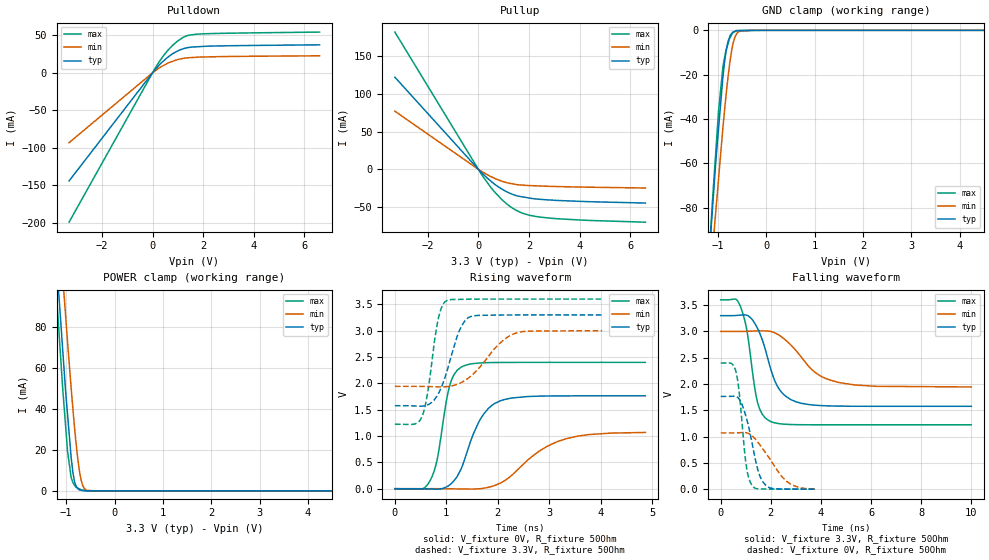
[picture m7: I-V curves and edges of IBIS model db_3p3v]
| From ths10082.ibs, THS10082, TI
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|   db_3p3v Model
[Model]   db_3p3v
Model_type   I/O
Polarity   Non-Inverting
Enable   Active-High
Vinl = 0.6
Vinh = 2
Vmeas = 1.65
Vref = 1.65
Cref = 30pF
Rref = 50
|   typ   min   max
C_comp   1.842e-12   1.833e-12   1.884e-12
[Voltage Range]   3.3   3   3.6
|Ambient Temperature   25   85   -40
|Junction Temperature
[Temperature Range]   27   125   -40
[Pullup Reference]   3.3   3   3.6
[Pulldown Reference]   0   0   0
[Power Clamp Reference]   3.3   3   3.6
[GND Clamp Reference]   0   0   0
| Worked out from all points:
|   slope of the pulldown table from 0 to 0.495 V, typ, clamps not added: 28 ohm
|   slope of the pullup table from 0 to 0.495 V, typ, clamps not added: 31.6 ohm
|   GND clamp passes 1 mA (typ) near -0.70 V on its own axis
|   POWER clamp passes 1 mA (typ) near -0.75 V on its own axis
|   falling waveform, V_fixture 3.3V, R_fixture 50Ohm: 20-80 % time 742ps typ, 1.28ns min, 446ps max; typ from 3.3 V to 1.58 V
|   rising waveform, V_fixture 0V, R_fixture 50Ohm: 20-80 % time 447ps typ, 848ps min, 252ps max; typ from 0 V to 1.76 V
|   rising waveform, V_fixture 3.3V, R_fixture 50Ohm: 20-80 % time 334ps typ, 575ps min, 209ps max; typ from 1.58 V to 3.3 V
|   falling waveform, V_fixture 0V, R_fixture 50Ohm: 20-80 % time 501ps typ, 943ps min, 292ps max; typ from 1.76 V to 0 V
[Pulldown]
|   Voltage   I(typ)   I(min)   I(max)
-3.3V     -144.5mA   -93.38mA   -199.6mA
154.8mV   6.391mA    3.9mA      9.041mA
424.8mV   15.59mA    9.622mA    22.52mA
630mV     21.64mA    13.42mA    30.96mA
1.008V    29.35mA    17.89mA    42.82mA
1.35V     33.32mA    19.96mA    49.36mA
1.836V    34.94mA    21.01mA    51.79mA
6.6V      37.38mA    22.72mA    54.4mA
[GND Clamp]
|   Voltage   I(typ)   I(min)   I(max)
-3.3V     -897.7mA   -838.9mA   -975.7mA
-1.234V   -118.3mA   -135.3mA   -121.5mA
-1.12V    -83.01mA   -102.4mA   -79.59mA
-1.065V   -66.19mA   -87.36mA   -61.92mA
-986.4mV  -44.52mA   -67.16mA   -36.62mA
-896.4mV  -21.17mA   -44.06mA   -16.6mA
-825mV    -8.688mA   -28.04mA   -8.718mA
-788.7mV  -4.936mA   -20.89mA   -5.997mA
-711mV    -1.339mA   -8.661mA   -1.849mA
-620.4mV  -156.6uA   -1.912mA   -275.6uA
-285mV    -71.48uA   -357.5nA   -115.2nA
6.6V      0A         0A         0A
[Pullup]
|   Voltage   I(typ)   I(min)   I(max)
-3.3V     122.1mA    77.06mA    181.9mA
172.8mV   -6.009mA   -3.688mA   -9.119mA
633.6mV   -19.54mA   -11.88mA   -29.75mA
918mV     -26.02mA   -15.65mA   -39.85mA
1.145V    -30.21mA   -17.93mA   -46.49mA
1.382V    -33.59mA   -19.49mA   -52.13mA
1.706V    -36.31mA   -20.85mA   -57.68mA
2.012V    -38.04mA   -21.53mA   -60.82mA
2.473V    -39.84mA   -22.12mA   -63.46mA
4.162V    -42.64mA   -23.56mA   -67.44mA
6.6V      -44.7mA    -24.77mA   -70.09mA
[POWER Clamp]
|   Voltage   I(typ)   I(min)   I(max)
-3.3V     939.7mA    939.4mA    959.6mA
-1.227V   122mA      157.3mA    105.9mA
-1.188V   107.9mA    143.9mA    91.32mA
-1.076V   70.24mA    106.6mA    51.39mA
-1.038V   57.3mA     93.74mA    39.49mA
-972mV    37.29mA    72.66mA    19.25mA
-861.3mV  9.013mA    40.08mA    4.173mA
-792mV    2.032mA    22.41mA    1.77mA
-726mV    538.1uA    9.65mA     988.8uA
-627mV    83.82uA    1.235mA    270.5uA
-399mV    53.18uA    2.449uA    499.6nA
6.6V      0A         0A         0A
[Ramp]
R_load = 50
|   typ   min   max
dV/dt_r   1.05825/4.45417e-10   0.642046/8.45388e-10   1.43893/2.51213e-10
dV/dt_f   1.0345/7.39471e-10   0.63381/1.27406e-09   1.42541/4.45762e-10
[Falling Waveform]
V_fixture = 3.3V
V_fixture_min = 3V
V_fixture_max = 3.6V
R_fixture = 50Ohm
|   Time   V(typ)   V(min)   V(max)
0s        3.3V       3V         3.6V
784ps     3.31V      3V         3.479V
1.06ns    3.304V     3.002V     2.978V
1.47ns    3.057V     3.009V     1.652V
1.952ns   2.356V     3.003V     1.296V
2.252ns   1.965V     2.951V     1.252V
2.752ns   1.716V     2.764V     1.23V
3.774ns   1.596V     2.218V     1.225V
4.712ns   1.579V     2.028V     1.224V
9.998ns   1.576V     1.944V     1.224V
[Rising Waveform]
V_fixture = 0V
V_fixture_min = 0V
V_fixture_max = 0V
R_fixture = 50Ohm
|   Time   V(typ)   V(min)   V(max)
0s        1.442nV    2.279nV    1.234nV
524ps     -1.324mV   201.4uV    -6.715mV
678ps     -5.487mV   230.6uV    140.5mV
824ps     -8.725mV   -95.2uV    561.4mV
1.066ns   72.5mV     -2.054mV   1.953V
1.304ns   412.9mV    -5.242mV   2.315V
1.662ns   1.318V     974.1uV    2.387V
2.054ns   1.669V     108.6mV    2.397V
3.174ns   1.762V     898.9mV    2.398V
4.872ns   1.764V     1.068V     2.398V
[Rising Waveform]
V_fixture = 3.3V
V_fixture_min = 3V
V_fixture_max = 3.6V
R_fixture = 50Ohm
|   Time   V(typ)   V(min)   V(max)
0s        1.576V     1.943V     1.224V
384ps     1.571V     1.943V     1.226V
526ps     1.567V     1.942V     1.363V
630ps     1.588V     1.939V     1.783V
844ps     1.801V     1.933V     3.224V
1.016ns   2.24V      1.938V     3.575V
1.246ns   2.98V      1.994V     3.594V
1.444ns   3.256V     2.111V     3.597V
2.3ns     3.298V     2.934V     3.6V
4.03ns    3.3V       2.999V     3.6V
[Falling Waveform]
V_fixture = 0V
V_fixture_min = 0V
V_fixture_max = 0V
R_fixture = 50Ohm
|   Time   V(typ)   V(min)   V(max)
0s        1.764V     1.07V      2.398V
430ps     1.766V     1.07V      2.391V
608ps     1.763V     1.071V     2.234V
740ps     1.712V     1.073V     1.828V
998ps     1.4V       1.074V     518.7mV
1.266ns   843.4mV    1.01V      62.51mV
1.524ns   302.9mV    867mV      5.273mV
1.806ns   69.82mV    681.5mV    2.016mV
2.632ns   2.175mV    148.9mV    256.4uV
3.776ns   274.6uV    2.765mV    134.8uV
